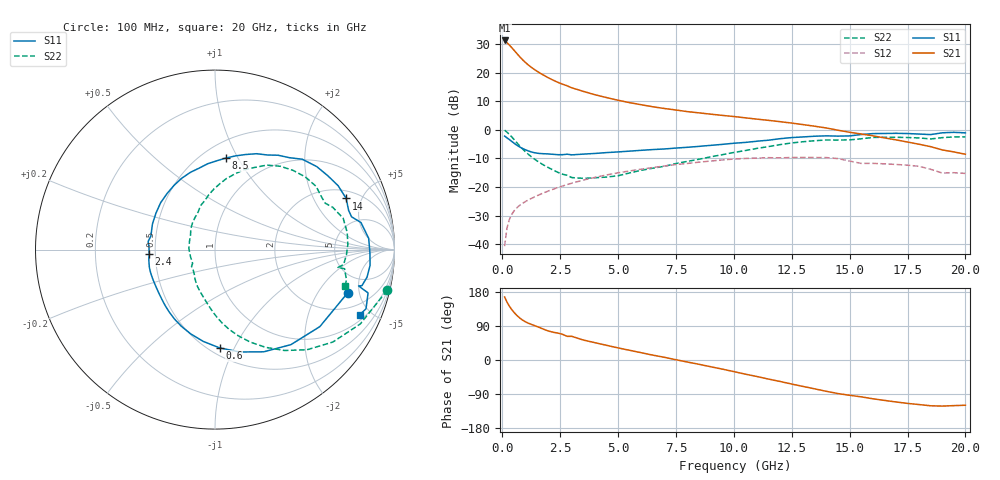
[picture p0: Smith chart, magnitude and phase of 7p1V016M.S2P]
! Infineon Technologies  Discrete & RF Semiconductors
! bfp620
! VCE =  1.0 V,  IC =  16 mA
! Common Emitter S-Parameters:  Sep 2002
# GHz  S  MA  R  50
!  f  S11  S21  S12  S22
! GHz  MAG  ANG  MAG  ANG  MAG  ANG  MAG  ANG
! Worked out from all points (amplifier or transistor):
!   59 points, 100 MHz to 20 GHz, reference 50 ohm
!   highest |S21| = 31.2 dB at 100 MHz (marker M1)
!   |S21| within 3 dB of that: start of sweep to 462 MHz
!   unconditionally stable (mu >= 1): 3.681 GHz to 10.11 GHz; 17.08 GHz to end of sweep
!   at 1 GHz: K = 0.63, MSG = 24.3 dB, |S12| = -25.1 dB
!   at 5.5 GHz: K = 1.04, MAG = 10.7 dB, |S12| = -14.4 dB
!   at 20 GHz: K = 1.41, MAG = -0.5 dB, |S12| = -15.2 dB
!   S11 on the Smith chart (normalised r, x): 100 MHz: 3.15, -3.83; 600 MHz: 0.56, -0.88; 2.4 GHz: 0.46, -0.02; 8.5 GHz: 0.64, +0.89; 14 GHz: 2.50, +3.71; 20 GHz: 1.29, -4.30
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0.1  0.7777 -18.0  36.3 166.3  0.0093 81.5  0.9857 -13.3
0.2  0.7248 -36.3  33.22 153.1  0.0191 72.8  0.9093 -27.1
0.3  0.6777 -51.4  30.31 142.5  0.0268 67.3  0.8345 -38.1
0.4  0.6309 -64.5  27.44 133.7  0.0329 62.9  0.7579 -47.4
0.5  0.5868 -76.4  24.68 126.1  0.038 59.3  0.683 -55.4
0.6  0.5482 -87.3  22.15 119.4  0.0424 56.6  0.6135 -62.6
0.7  0.5159 -97.2  19.91 113.6  0.0462 54.4  0.5517 -69.1
0.8  0.4892 -105.9  17.98 108.6  0.0496 52.9  0.4982 -74.8
0.9  0.4668 -113.6  16.35 104.3  0.0528 51.8  0.4527 -79.8
1.1  0.4315 -126.2  13.8 97.8  0.0588 50.4  0.381 -87.9
1.4  0.3974 -141.2  11.21 90.6  0.0676 49.2  0.3063 -97.6
1.8  0.382 -157.9  8.913 80.9  0.0797 47.6  0.2411 -111.4
2.4  0.3676 -176.6  6.744 71.0  0.0981 44.6  0.1806 -129.5
3.5  0.3765 157.8  4.688 52.7  0.1327 36.7  0.142 -164.5
5  0.4111 130.5  3.282 31.9  0.1776 23.8  0.1577 149.8
7  0.4626 100.9  2.355 7.1  0.2333 5.2  0.2307 113.9
8.5  0.5138 83.2  1.975 -11.4  0.2724 -10.1  0.3064 96.6
10.5  0.6025 61.0  1.617 -37.4  0.3162 -33.5  0.4348 75.4
13.5  0.773 27.4  1.154 -76.2  0.328 -68.4  0.6453 39.0
14  0.7844 21.3  1.075 -82.7  0.3275 -75.1  0.6646 32.0
17  0.8685 -5.8  0.668 -110.7  0.2483 -99.5  0.7407 2.2
20  0.8847 -24.2  0.375 -119.4  0.1732 -110.5  0.7529 -15.8
